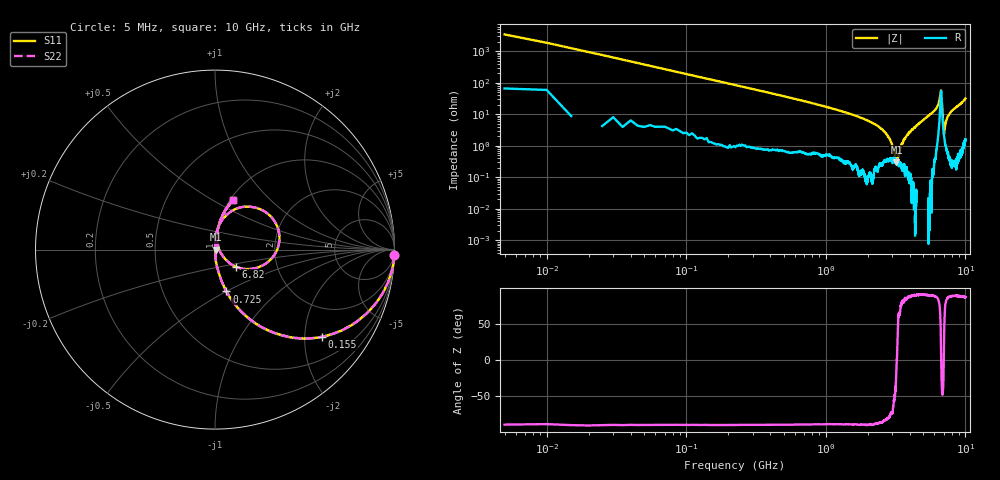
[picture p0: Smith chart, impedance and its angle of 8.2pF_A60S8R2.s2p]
! Amotech Co.,Ltd.
! http://www.amotech.co.kr/
! Part Number: A60S8R2
! These Parameters are Measured in Series Mode Connection
! Operation Temp=25[degC], DC Bias Voltage=0[V]
! Freq. Start=5[MHz] Stop=10[GHz], 2000[Steps]
! Date: Monday, July 13, 2020, 01:57:41
# GHZ S RI R 50.000000
!Freq.(Hz) S11(Real) S11(Imag) S21(Real) S21(Imag) S12(Real) S12(Imag) S22(Real) S22(Imag)
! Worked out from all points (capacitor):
!   2000 points, 5 MHz to 10 GHz, reference 50 ohm
!   read as one part in series: C = 8.46 pF near 55 MHz
!   lowest |Z| = 302 mohm at 3.205 GHz (marker M1)
!   series resonance near 3.223 GHz, so ESL is about 290 pH
!   S11 on the Smith chart (normalised r, x): 5 MHz: 2, -67; 155 MHz: 1.02, -2.44; 725 MHz: 1.01, -0.50; 6.82 GHz: 1.23, -0.24; 10 GHz: 1.03, +0.63
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0.005  0.9985 -0.0297  0.00146 0.0297  0.00146 0.0297  0.9985 -0.0297
0.075  0.8591 -0.3409  0.1409 0.3409  0.1409 0.3409  0.8591 -0.3409
0.155  0.5963 -0.4857  0.4037 0.4857  0.4037 0.4857  0.5963 -0.4857
0.36  0.2171 -0.4052  0.7829 0.4052  0.7829 0.4052  0.2171 -0.4052
0.725  0.0633 -0.2329  0.9367 0.2329  0.9367 0.2329  0.0633 -0.2329
1.675  0.0095 -0.0848  0.9905 0.0848  0.9905 0.0848  0.0095 -0.0848
2.71  0.00401 -0.0238  0.996 0.0238  0.996 0.0238  0.00401 -0.0238
2.945  0.00407 -0.0121  0.9959 0.0121  0.9959 0.0121  0.00407 -0.0121
3.205  0.00292 -0.000737  0.9971 0.000737  0.9971 0.000737  0.00292 -0.000737
3.34  0.00271 0.0049  0.9973 -0.0049  0.9973 -0.0049  0.00271 0.0049
3.475  0.00272 0.0104  0.9973 -0.0104  0.9973 -0.0104  0.00272 0.0104
3.81  0.00189 0.0211  0.9981 -0.0211  0.9981 -0.0211  0.00189 0.0211
5.005  0.00366 0.066  0.9963 -0.066  0.9963 -0.066  0.00366 0.066
6.35  0.0483 0.1765  0.9517 -0.1765  0.9517 -0.1765  0.0483 0.1765
6.58  0.184 0.2395  0.816 -0.2395  0.816 -0.2395  0.184 0.2395
6.67  0.3469 0.1295  0.6531 -0.1295  0.6531 -0.1295  0.3469 0.1295
6.82  0.1151 -0.0951  0.8849 0.0951  0.8849 0.0951  0.1151 -0.0951
6.97  0.0282 -0.0114  0.9718 0.0114  0.9718 0.0114  0.0282 -0.0114
7.025  0.021 0.00824  0.979 -0.00824  0.979 -0.00824  0.021 0.00824
7.435  0.0121 0.0788  0.9879 -0.0788  0.9879 -0.0788  0.0121 0.0788
8.335  0.0242 0.1457  0.9758 -0.1457  0.9758 -0.1457  0.0242 0.1457
10  0.101 0.2772  0.899 -0.2772  0.899 -0.2772  0.101 0.2772
